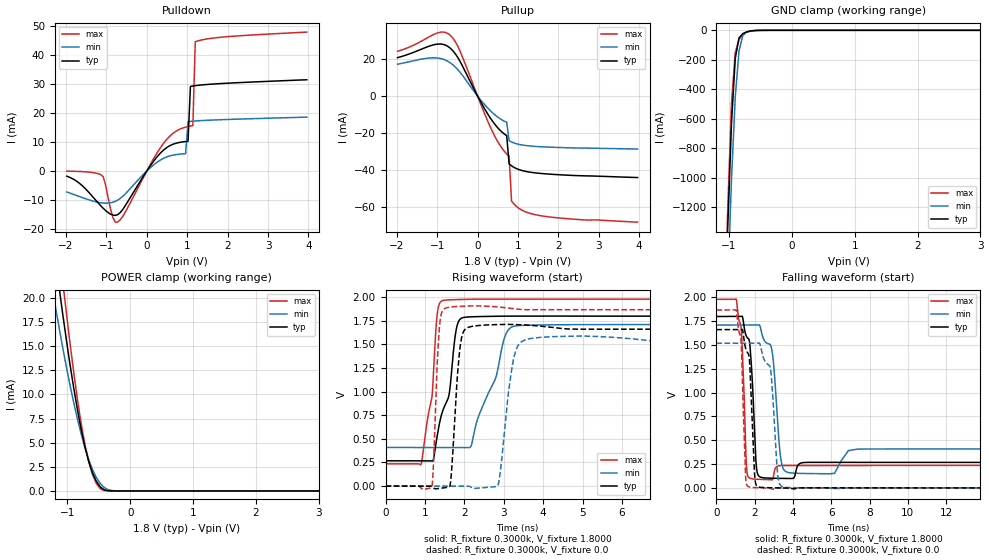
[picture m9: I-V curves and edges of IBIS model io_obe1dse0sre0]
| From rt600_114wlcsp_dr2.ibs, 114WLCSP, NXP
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[Model] io_obe1dse0sre0
|   Model io_obe1dse0sre0
| Library cells for typ/min/max conditions are connected as defined below:
|  pad - External Pad
|  ipp_do - Core Input
|  ipp_obe - Output Buffer Enable
|  REFH3V3 - vdd1v8
|  REFL3V3 - REFL3V3
|  gnde - gnde
|  ipp_ina235_3v - NC
|  ipp_ina40_3v - NC
|  ipp_ina_mux - NC
|  ipp_ind - NC
|  ipp_ind_1p8v - NC
|  ipp_ind_3v - NC
|  vdd - vdd
|  vdd1v8 - vdd1v8
|  vdda - vdde3v3
|  vdde3v3 - vdde3v3
| All other pins connected to ground
Model_type I/O
Polarity   Non-Inverting
Enable   Active-High
Vinl =   0.5400V
Vinh =   1.2600V
Vmeas =  0.9000V
Cref =   25.0000pF
Rref =   0.5000k
Vref =   0.0V
C_comp   2.2458pF   2.1703pF   2.3896pF
[Temperature Range]   25.0000   0.1250k   -40.0000
[Voltage Range]   1.8000V   1.7100V   1.9800V
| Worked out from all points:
|   slope of the pulldown table from 0 to 0.27 V, typ, clamps not added: 52.6 ohm
|   slope of the pullup table from 0 to 0.27 V, typ, clamps not added: 26.1 ohm
|   GND clamp passes 1 mA (typ) near -0.57 V on its own axis
|   POWER clamp passes 1 mA (typ) near -0.54 V on its own axis
|   rising waveform, R_fixture 0.3000k, V_fixture 1.8000: 20-80 % time 411ps typ, 638ps min, 252ps max; typ from 0.268 V to 1.8 V
|   rising waveform, R_fixture 0.3000k, V_fixture 0.0: 20-80 % time 153ps typ, 241ps min, 107ps max; typ from 0 V to 1.66 V
|   falling waveform, R_fixture 0.3000k, V_fixture 1.8000: 20-80 % time 242ps typ, 309ps min, 192ps max; typ from 1.8 V to 0.268 V
|   falling waveform, R_fixture 0.3000k, V_fixture 0.0: 20-80 % time 218ps typ, 289ps min, 175ps max; typ from 1.66 V to 0 V
[Pulldown]
|Voltage   I(typ)   I(min)   I(max)
-1.98V    -1.78mA    -7.2mA     -50uA
-1.08V    -12.8mA    -11.03mA   -1.913mA
-840mV    -15.17mA   -10.75mA   -15.99mA
-720mV    -15.01mA   -10.02mA   -17.56mA
300mV     5.617mA    3.457mA    7.23mA
600mV     8.925mA    5.324mA    12.39mA
960mV     10.14mA    5.952mA    15.11mA
1.02V     10.21mA    16.97mA    15.31mA
1.08V     29.1mA     17.07mA    15.48mA
1.14V     29.25mA    17.15mA    15.61mA
1.2V      29.37mA    17.22mA    44.52mA
3.96V     31.41mA    18.55mA    47.82mA
[Pullup]
|Voltage   I(typ)   I(min)   I(max)
-1.98V    20.86mA    17.3mA     24.34mA
-960mV    28.24mA    20.54mA    34.46mA
-780mV    27.49mA    19.36mA    34.38mA
-600mV    24.29mA    16.74mA    31.09mA
-420mV    18.25mA    12.55mA    23.63mA
360mV     -13.31mA   -8.861mA   -18.88mA
720mV     -21.45mA   -14.21mA   -31.33mA
780mV     -36.76mA   -24.2mA    -32.57mA
840mV     -37.8mA    -24.87mA   -56.93mA
1.02V     -39.81mA   -26.15mA   -60.8mA
1.8V      -42.33mA   -27.69mA   -65.55mA
3.96V     -44.16mA   -28.7mA    -68.35mA
[GND_clamp]
|Voltage   I(typ)   I(min)   I(max)
-1.98V    -17.57A    -17.55A    -18.13A
-1.08V    -2.185A    -2.567A    -2.121A
-1.02V    -1.339A    -1.74A     -1.223A
-960mV    -630.1mA   -1.012A    -499.4mA
-900mV    -189.5mA   -452.2mA   -152mA
-840mV    -51.34mA   -139.9mA   -62.86mA
-780mV    -22.28mA   -35.54mA   -26.58mA
-720mV    -10.62mA   -11.15mA   -13.18mA
-600mV    -1.527mA   -2.152mA   -2.249mA
-480mV    -85.63uA   -243.9uA   -63.17uA
3.96V     0A         0A         0A
[POWER_clamp]
|Voltage   I(typ)   I(min)   I(max)
-1.98V    66.18mA    51.42mA    77.85mA
-1.26V    27.66mA    21.8mA     33.09mA
-1.2V     24.56mA    19.48mA    29.34mA
-1.14V    21.54mA    17.24mA    25.67mA
-1.08V    18.63mA    15.07mA    22.11mA
-1.02V    15.84mA    13mA       18.69mA
-840mV    8.434mA    7.464mA    9.5mA
-720mV    4.556mA    4.476mA    4.785mA
-600mV    1.876mA    2.218mA    1.703mA
-540mV    1.008mA    1.402mA    786.9uA
-420mV    135uA      383.7uA    43.39uA
3.96V     0A         0A         0A
[Ramp]
| variable   typ   min   max
dV/dt_r  0.6454/0.1807n   0.4661/0.2714n   0.8344/0.1289n
dV/dt_f  0.7379/0.3469n   0.4996/0.4270n   0.4742/0.3066n
R_load = 50.0000
[Rising Waveform]
R_fixture= 0.3000k
V_fixture= 1.8000
V_fixture_min= 1.7100
V_fixture_max= 1.9800
|time   V(typ)   V(min)   V(max)
0s        267.9mV    408.9mV    235.9mV
897.5ps   267.9mV    408.9mV    227.6mV
1.202ns   268.4mV    408.9mV    1.089V
1.371ns   670.9mV    408.9mV    1.937V
1.609ns   964.3mV    408.9mV    1.973V
1.828ns   1.718V     408.9mV    1.976V
2.264ns   1.794V     596.7mV    1.98V
3.144ns   1.8V       1.668V     1.981V
4.652ns   1.8V       1.71V      1.98V
500ns     1.8V       1.71V      1.98V
[Rising Waveform]
R_fixture= 0.3000k
V_fixture= 0.0
V_fixture_min= 0.0
V_fixture_max= 0.0
|time   V(typ)   V(min)   V(max)
0s        65.01nV    1.918uV    111.1nV
1.176ns   -5.715mV   1.908uV    -8.332mV
1.375ns   -24.64mV   1.834uV    1.719V
1.628ns   -4.041mV   1.504uV    1.895V
1.904ns   1.511V     695nV      1.904V
2.22ns    1.694V     -22.44mV   1.909V
2.854ns   1.711V     10.72mV    1.897V
3.404ns   1.709V     1.512V     1.871V
4.957ns   1.662V     1.589V     1.868V
500ns     1.662V     1.519V     1.868V
[Falling Waveform]
R_fixture= 0.3000k
V_fixture= 1.8000
V_fixture_min= 1.7100
V_fixture_max= 1.9800
|time   V(typ)   V(min)   V(max)
0s        1.8V       1.71V      1.98V
1.033ns   1.8V       1.71V      1.982V
1.364ns   1.796V     1.71V      1.391V
1.62ns    1.576V     1.71V      140mV
1.781ns   1.423V     1.71V      99.65mV
2.115ns   179.9mV    1.709V     90.87mV
2.878ns   101.8mV    1.468V     84.22mV
3.487ns   99.95mV    203.5mV    235.6mV
5.648ns   268.3mV    148.9mV    236mV
500ns     267.9mV    408.9mV    235.9mV
[Falling Waveform]
R_fixture= 0.3000k
V_fixture= 0.0
V_fixture_min= 0.0
V_fixture_max= 0.0
|time   V(typ)   V(min)   V(max)
0s        1.662V     1.519V     1.868V
1.048ns   1.662V     1.519V     1.859V
1.293ns   1.662V     1.519V     1.528V
1.575ns   1.438V     1.519V     37.7mV
1.73ns    1.327V     1.519V     9.143mV
2.04ns    56.01mV    1.518V     2.742mV
2.933ns   1.597mV    995.7mV    -13.09mV
3.327ns   1.183mV    32.19mV    581.8uV
6.392ns   202.5uV    -6.117mV   16.29uV
500ns     1.116uV    3.176uV    679.6nV
